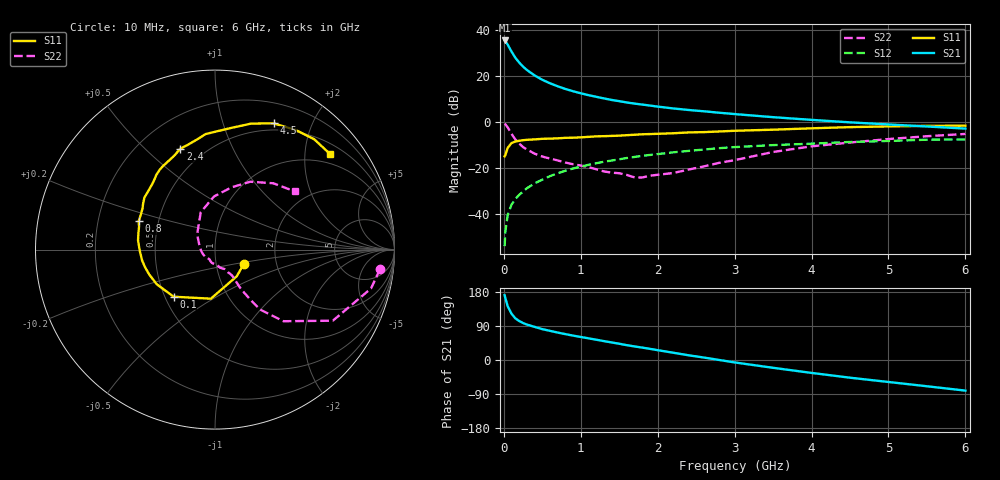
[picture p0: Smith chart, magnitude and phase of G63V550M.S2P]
! SIEMENS Small Signal Semiconductors
! BFG193
! Si NPN RF Bipolar Junction Transistor in SOT223
! VCE = 3.5 V  IC = 50 mA
! Common Emitter S-Parameters:  August  1996
# GHz  S  MA  R  50
!  f  S11  S21  S12  S22
! GHz  MAG  ANG  MAG  ANG  MAG  ANG  MAG  ANG
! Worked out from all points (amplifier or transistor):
!   36 points, 10 MHz to 6 GHz, reference 50 ohm
!   highest |S21| = 35.5 dB at 10 MHz (marker M1)
!   |S21| within 3 dB of that: start of sweep to 69.62 MHz
!   unconditionally stable (mu >= 1): 431.4 MHz to 2.343 GHz
!   at 250 MHz: K = 0.93, MSG = 27.2 dB, |S12| = -30.2 dB
!   at 1.4 GHz: K = 1.05, MAG = 11.9 dB, |S12| = -16.8 dB
!   at 6 GHz: K = 0.90, MSG = 2.4 dB, |S12| = -7.6 dB
!   S11 on the Smith chart (normalised r, x): 10 MHz: 1.36, -0.23; 100 MHz: 0.55, -0.33; 800 MHz: 0.39, +0.16; 2.4 GHz: 0.37, +0.65; 4.5 GHz: 0.42, +1.48; 6 GHz: 0.74, +2.59
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0.01  0.1792 -27.3  59.4 170.9  0.002 85.0  0.9255 -6.8
0.02  0.1919 -50.9  57.17 163.1  0.0042 76.9  0.8959 -14.0
0.05  0.2744 -94.8  48.22 142.0  0.0095 70.2  0.7669 -31.1
0.1  0.3493 -131.3  34.02 122.1  0.016 67.7  0.5519 -46.3
0.15  0.3779 -149.4  24.93 109.8  0.0212 66.8  0.4173 -53.1
0.2  0.392 -159.3  19.63 102.9  0.0262 68.2  0.3407 -54.8
0.25  0.4028 -166.4  16.02 97.5  0.0308 68.2  0.2849 -56.0
0.3  0.4108 -171.8  13.54 93.5  0.0363 69.8  0.2529 -56.7
0.4  0.4195 -179.3  10.3 87.4  0.0465 69.6  0.2052 -56.6
0.5  0.432 173.1  8.288 81.5  0.0558 68.4  0.1775 -56.4
0.6  0.4363 168.0  6.961 76.9  0.0666 67.7  0.1609 -57.7
0.7  0.4419 163.3  5.99 72.4  0.0768 66.4  0.1464 -60.0
0.8  0.4538 159.4  5.236 68.3  0.0872 64.1  0.1317 -62.2
1.1  0.4759 147.3  3.844 57.2  0.1172 59.1  0.1047 -74.2
1.3  0.4925 140.2  3.266 49.9  0.1368 54.9  0.0845 -84.2
1.6  0.518 130.4  2.659 39.1  0.1653 48.0  0.0706 -109.8
2.2  0.5697 113.6  1.978 19.3  0.2192 34.4  0.0778 -175.1
2.4  0.5942 109.0  1.83 12.5  0.2354 30.2  0.0923 162.2
3.5  0.6818 82.9  1.276 -20.6  0.3146 3.0  0.2233 110.8
4.5  0.7755 65.1  0.984 -46.7  0.3688 -17.0  0.3586 75.2
5.5  0.8267 48.1  0.8 -69.3  0.4134 -40.3  0.4919 48.7
6  0.8336 39.6  0.721 -80.8  0.4182 -53.6  0.5509 36.0
